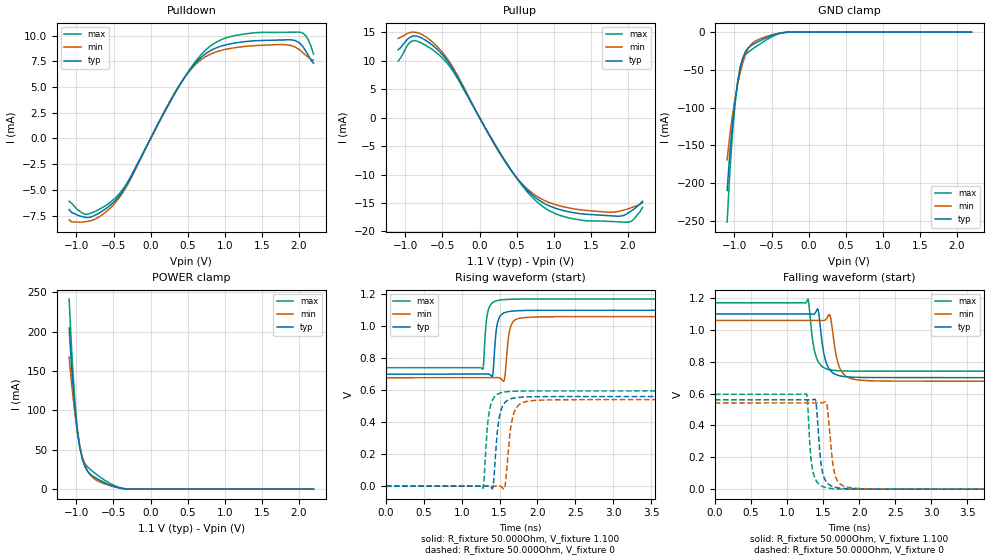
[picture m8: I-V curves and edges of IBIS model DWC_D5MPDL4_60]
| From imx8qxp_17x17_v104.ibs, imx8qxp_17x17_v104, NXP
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[Model] DWC_D5MPDL4_60
Model_type   I/O
Polarity   Non-Inverting
Enable   Active-High
C_comp   1.572pF   1.476pF   1.691pF
C_comp_pullup   368.743fF   352.502fF   369.274fF
C_comp_pulldown 1.168pF   1.095pF   1.338pF
Vinh = 404.000mV
Vinl = 224.000mV
Vmeas = 314.000mV
Vref = 314.000mV
Rref = 50Ohms
Cref = 0pF
[Model Spec]
Vinh   404.000mV   393.000mV   424.000mV
Vinl   224.000mV   213.000mV   244.000mV
Vmeas   314.000mV   303.000mV   334.000mV
Vref   314.000mV   303.000mV   334.000mV
D_overshoot_ampl_h 0.35 NA   NA
D_overshoot_ampl_l 0.35 NA   NA
D_overshoot_area_l 800.000p NA   NA
D_overshoot_area_h 800.000p NA   NA
[Receiver Thresholds]
Vcross_low = 219.000mV
Vcross_high = 409.000mV
Vdiff_ac = 140.000mV
Vdiff_dc = 140.000mV
Tdiffslew_ac = 10.000ns
[Temperature Range]   25.000   125.000   -40.000
[Voltage Range]   1.100V   1.060V   1.170V
[GND Clamp Reference]   0.00V   0.00V   0.00V
[Pulldown Reference]   0.00V   0.00V   0.00V
[POWER Clamp Reference]   1.100V   1.060V   1.170V
[Pullup Reference]   1.100V   1.060V   1.170V
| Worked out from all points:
|   slope of the pulldown table from 0 to 0.165 V, typ, clamps not added: 72.2 ohm
|   slope of the pullup table from 0 to 0.165 V, typ, clamps not added: 43.3 ohm
|   GND clamp passes 1 mA (typ) near -0.36 V on its own axis
|   POWER clamp passes 1 mA (typ) near -0.39 V on its own axis
|   rising waveform, R_fixture 50.000Ohm, V_fixture 1.100: 20-80 % time 47.7ps typ, 53.2ps min, 45.6ps max; typ from 0.7 V to 1.1 V
|   rising waveform, R_fixture 50.000Ohm, V_fixture 0: 20-80 % time 69.6ps typ, 78.8ps min, 63.9ps max; typ from 0 V to 0.561 V
|   falling waveform, R_fixture 50.000Ohm, V_fixture 1.100: 20-80 % time 94.8ps typ, 104ps min, 87.6ps max; typ from 1.1 V to 0.7 V
|   falling waveform, R_fixture 50.000Ohm, V_fixture 0: 20-80 % time 69ps typ, 77.8ps min, 62.6ps max; typ from 0.561 V to 0 V
[GND Clamp]
-1.099V   -209.8mA   -169.1mA   -251.7mA
-1.064V   -162.7mA   -137.8mA   -187.8mA
-1.028V   -123.6mA   -111mA     -135.8mA
-992.7mV  -92.04mA   -88.31mA   -95.63mA
-957.3mV  -67.05mA   -69.29mA   -65.81mA
-921.8mV  -47.73mA   -53.39mA   -45.6mA
-886.4mV  -33.92mA   -40.26mA   -34.72mA
-815.5mV  -20.84mA   -22.1mA    -26.75mA
-673.6mV  -12.32mA   -9.665mA   -16.87mA
-460.9mV  -3.34mA    -2.899mA   -4.539mA
-319.1mV  -390.9uA   -567.4uA   -395.4uA
2.198V    38.31nA    663.5nA    7.807nA
[Power Clamp]
-1.098V   204.7mA    167.9mA    241.5mA
-1.063V   153.5mA    132.2mA    175.1mA
-1.027V   110.2mA    101.3mA    120.2mA
-991.8mV  76.87mA    75.61mA    80.19mA
-956.4mV  53.56mA    55.87mA    54.83mA
-920.9mV  38.25mA    41.27mA    40.22mA
-885.5mV  28.61mA    30.83mA    32.49mA
-814.5mV  19.18mA    18.23mA    25.18mA
-743.6mV  14.55mA    12.13mA    19.82mA
-495.5mV  3.463mA    3.102mA    4.838mA
-318.2mV  225.2uA    399.5uA    248.6uA
2.199V    -19.18nA   -668.9nA   -2.437nA
[Pulldown]
-1.099V   -6.9mA     -7.9mA     -6.1mA
-850.9mV  -7.684mA   -8.055mA   -7.361mA
-638.2mV  -6.993mA   -7.334mA   -6.66mA
-425.5mV  -5.595mA   -5.778mA   -5.403mA
-283.6mV  -4.006mA   -4.143mA   -3.899mA
354.5mV   4.731mA    4.788mA    4.708mA
567.3mV   6.992mA    6.899mA    7.114mA
780mV     8.411mA    8.095mA    8.829mA
1.17V     9.308mA    8.851mA    10.04mA
1.915V    9.567mA    8.977mA    10.33mA
2.092V    8.505mA    8.1mA      9.994mA
2.198V    7.3mA      7.6mA      8.2mA
[Pullup]
-1.098V   11.9mA     13.93mA    9.915mA
-956.4mV  13.95mA    14.86mA    13mA
-885.5mV  14.35mA    15.02mA    13.54mA
-708.2mV  13.41mA    14.04mA    12.55mA
-495.5mV  10.98mA    11.38mA    10.39mA
-318.2mV  7.652mA    7.925mA    7.347mA
320mV     -7.156mA   -7.256mA   -7.073mA
745.5mV   -13.96mA   -13.58mA   -14.44mA
1.029V    -15.94mA   -15.31mA   -16.9mA
1.455V    -17mA      -16.32mA   -18.14mA
2.022V    -16.62mA   -15.97mA   -18.35mA
2.199V    -14.7mA    -14.99mA   -15.78mA
[Ramp]
R_load=50.000Ohm
dV/dt_r   288.120mV/59.000ps  276.899mV/67.000ps  307.470mV/56.000ps
dV/dt_f   288.090mV/83.000ps  276.899mV/92.000ps  307.440mV/76.000ps
[Rising waveform]
R_fixture=50.000Ohm
V_fixture=1.100
V_fixture_min=1.060
V_fixture_max=1.170
0s        700.5mV    678.3mV    741mV
1.283ns   700.5mV    678.3mV    732.2mV
1.333ns   701.1mV    678.3mV    1.06V
1.403ns   682.7mV    678.2mV    1.145V
1.464ns   999.3mV    679.4mV    1.16V
1.564ns   1.085V     664.1mV    1.167V
1.614ns   1.091V     916.2mV    1.168V
1.644ns   1.093V     995.2mV    1.169V
1.844ns   1.099V     1.055V     1.17V
10ns      1.1V       1.06V      1.17V
[Rising waveform]
R_fixture=50.000Ohm
V_fixture=0
0s        158.6nV    4.671uV    25.1nV
1.283ns   -34.17uV   2.852uV    -13.38mV
1.333ns   319.2uV    19.62uV    339.4mV
1.373ns   548.4uV    -22.82uV   488.1mV
1.413ns   -7.626mV   -108uV     544.2mV
1.494ns   425.4mV    1.333mV    580.2mV
1.584ns   529.6mV    49.65mV    590.5mV
1.684ns   551.1mV    450.8mV    593.9mV
1.904ns   559.3mV    533.7mV    595.8mV
10ns      560.9mV    541.3mV    595.9mV
[Falling waveform]
R_fixture=50.000Ohm
V_fixture=1.100
V_fixture_min=1.060
V_fixture_max=1.170
0s        1.1V       1.06V      1.17V
1.293ns   1.1V       1.06V      1.194V
1.363ns   1.099V     1.06V      911.5mV
1.423ns   1.133V     1.06V      809.2mV
1.514ns   844.8mV    1.06V      762.2mV
1.594ns   749.1mV    1.094V     749.8mV
1.664ns   722.6mV    883mV      745.4mV
1.784ns   707.8mV    722.8mV    742.4mV
2.095ns   701.3mV    682mV      740.8mV
10ns      700.5mV    678.3mV    741mV
[Falling waveform]
R_fixture=50.000Ohm
V_fixture=0
0s        560.8mV    541.3mV    595.8mV
1.273ns   560.8mV    541.3mV    595.7mV
1.363ns   562mV      541.3mV    103.9mV
1.403ns   542.8mV    541.3mV    53.75mV
1.484ns   123.7mV    541.9mV    18.5mV
1.554ns   40.55mV    528mV      8.243mV
1.594ns   25.25mV    349.6mV    5.299mV
1.684ns   10.28mV    65.95mV    2.06mV
1.945ns   1.092mV    5.777mV    192uV
10ns      572.2nV    4.699uV    216.4nV
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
